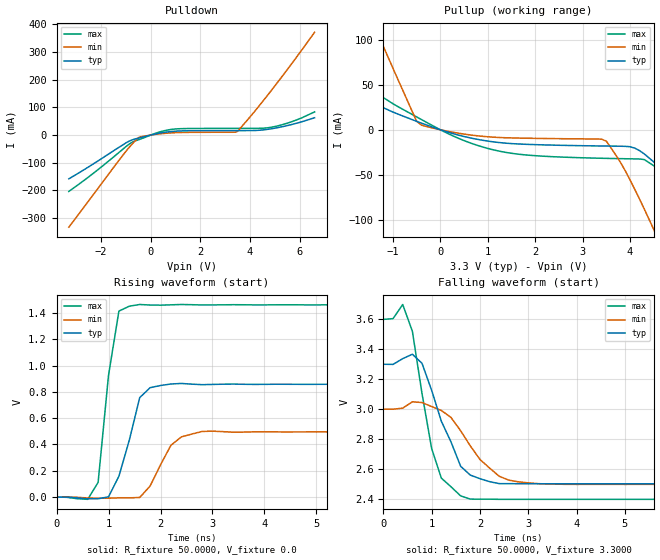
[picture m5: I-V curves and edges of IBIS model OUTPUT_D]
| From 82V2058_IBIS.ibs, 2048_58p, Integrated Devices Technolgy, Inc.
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|   Model OUTPUT_D
[Model]   OUTPUT_D
Model_type   Output
Polarity   Non-Inverting
Vmeas =   1.65V
C_comp   2.6600pF   2.5500pF   2.7500pF
[Temperature Range]   25.0000   85.0000   -40.0000
[Voltage Range]   3.3000V   3.0000V   3.6000V
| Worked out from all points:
|   slope of the pulldown table from 0 to 0.495 V, typ, clamps not added: 54.8 ohm
|   slope of the pullup table from 0 to 0.495 V, typ, clamps not added: 66.6 ohm
|   rising waveform, R_fixture 50.0000, V_fixture 0.0: 20-80 % time 347ps typ, 390ps min, 255ps max; typ from 0 V to 0.858 V
|   falling waveform, R_fixture 50.0000, V_fixture 3.3000: 20-80 % time 564ps typ, 729ps min, 422ps max; typ from 3.3 V to 2.5 V
[Pulldown]
|Voltage   I(typ)   I(min)   I(max)
-3.3V     -158.2mA   -332.9mA   -203.7mA
-2.3V     -103.5mA   -213.8mA   -137.3mA
-1V       -28.38mA   -58.79mA   -41.86mA
-800mV    -19.13mA   -37.45mA   -28.62mA
-500mV    -11.28mA   -9.712mA   -17.25mA
300mV     6.013mA    3.742mA    9.709mA
900mV     13.39mA    8.261mA    21.26mA
3.5V      16.11mA    13.39mA    24.2mA
4.3V      16.95mA    98.13mA    24.36mA
4.9V      23.26mA    166.1mA    29.01mA
5.7V      38.59mA    260.8mA    48.98mA
6.6V      62.62mA    371.4mA    83.82mA
[Pullup]
|Voltage   I(typ)   I(min)   I(max)
-3.2V     73.64mA    336.4mA    101.7mA
-1.4V     29.1mA     116.4mA    42.31mA
-500mV    9.336mA    9.491mA    14.26mA
700mV     -9.82mA    -6.225mA   -15.9mA
1.7V      -15.93mA   -9.306mA   -27.44mA
3.4V      -18.02mA   -10.43mA   -31.65mA
3.7V      -18.22mA   -28.03mA   -31.98mA
4.1V      -20.39mA   -66.11mA   -32.36mA
4.5V      -35.71mA   -110.7mA   -39.88mA
5.5V      -90.83mA   -229.5mA   -107.6mA
5.9V      -113.8mA   -277.5mA   -136.6mA
6.6V      -152.8mA   -360.5mA   -185.8mA
[Ramp]
| variable   typ   min   max
dV/dt_r   0.5147/0.2741n   0.2974/0.3846n   0.8772/0.2180n
dV/dt_f   0.4794/0.4931n   0.3018/0.7183n   0.7218/0.3760n
R_load =   50.0000
[Rising Waveform]
R_fixture=   50.0000
V_fixture=   0.0
V_fixture_min=  0.0
V_fixture_max=  0.0
|time   V(typ)   V(min)   V(max)
0s        0V         0V         0V
800ps     -12.87mV   -9.484mV   111.5mV
1ns       1.403mV    -8.523mV   926.4mV
1.2ns     158.6mV    -6.342mV   1.415V
1.4ns     433.2mV    -6.197mV   1.452V
1.6ns     756.3mV    -3.369mV   1.465V
1.8ns     832.2mV    83.63mV    1.461V
2.2ns     860.3mV    393.7mV    1.462V
2.8ns     855mV      498.9mV    1.461V
10ns      857.9mV    495.6mV    1.462V
[Falling Waveform]
R_fixture=   50.0000
V_fixture=   3.3000
V_fixture_min=  3.0000
V_fixture_max=  3.6000
|time   V(typ)   V(min)   V(max)
0s        3.3V       3V         3.6V
400ps     3.337V     3.006V     3.7V
600ps     3.367V     3.049V     3.521V
800ps     3.306V     3.044V     3.104V
1ns       3.125V     3.017V     2.736V
1.2ns     2.919V     2.991V     2.539V
1.6ns     2.618V     2.856V     2.42V
2.2ns     2.515V     2.606V     2.398V
2.8ns     2.501V     2.514V     2.397V
10ns      2.501V     2.497V     2.397V
